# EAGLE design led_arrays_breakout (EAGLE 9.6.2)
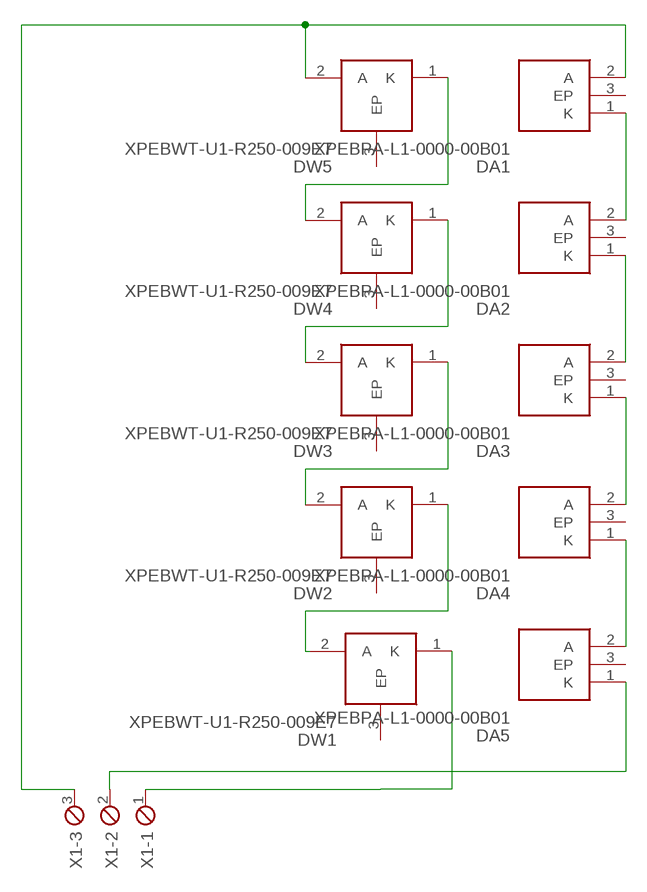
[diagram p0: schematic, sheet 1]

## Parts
DA1  XPEBPA-L1-0000-00B01  [XPEBPAL1000000B01]
DA2  XPEBPA-L1-0000-00B01  [XPEBPAL1000000B01]
DA3  XPEBPA-L1-0000-00B01  [XPEBPAL1000000B01]
DA4  XPEBPA-L1-0000-00B01  [XPEBPAL1000000B01]
DA5  XPEBPA-L1-0000-00B01  [XPEBPAL1000000B01]
DW1  XPEBWT-U1-R250-009E7  [XPEWHTL1000000E01]
DW2  XPEBWT-U1-R250-009E7  [XPEWHTL1000000E01]
DW3  XPEBWT-U1-R250-009E7  [XPEWHTL1000000E01]
DW4  XPEBWT-U1-R250-009E7  [XPEWHTL1000000E01]
DW5  XPEBWT-U1-R250-009E7  [XPEWHTL1000000E01]
X1  MPT3  [3POL254]

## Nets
N$1: DW4.2(A) DW5.1(K)
N$2: DW3.2(A) DW4.1(K)
N$3: DW2.2(A) DW3.1(K)
N$4: DW1.2(A) DW2.1(K)
N$5: DA5.1(K) X1.2
N$6: DW1.1(K) X1.1
N$9: DA1.2(A) DW5.2(A) X1.3
N$24: DA1.1(K) DA2.2(A)
N$25: DA2.1(K) DA3.2(A)
N$26: DA3.1(K) DA4.2(A)
N$27: DA4.1(K) DA5.2(A)
Unconnected: DA1.3(EP) DA2.3(EP) DA3.3(EP) DA4.3(EP) DA5.3(EP) DW1.3(EP) DW2.3(EP) DW3.3(EP) DW4.3(EP) DW5.3(EP)

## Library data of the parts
DA1-DA5 = SamacSys_Parts:XPEBPA-L1-0000-00B01: Cree XPEBPA-L1-0000-00B01, XLamp XP-E2 Series PC Amber LED, 595 nm, Clear, Dome Lens SMD Package Source: Datasheet; DESCRIPTION: Cree XPEBPA-L1-0000-00B01, XLamp XP-E2 Series PC Amber LED, 595 nm, Clear, Dome Lens SMD Package; HEIGHT: 2.53mm; MANUFACTURER_NAME: Wolfspeed; MANUFACTURER_PART_NUMBER: XPEBPA-L1-0000-00B01; MOUSER_PART_NUMBER: 941-XPEBPAL10000B01; MOUSER_PRICE-STOCK: https://www.mouser.co.uk/ProductDetail/Cree-Inc/XPEBPA-L1-0000-00B01?qs=odi%2FggezlBvEJ61b2kTHEA%3D%3D
DW1-DW5 = SamacSys_Parts:XPEBWT-U1-R250-009E7: Cree XPEBWT-U1-R250-009E7, XLamp XP-E2 Series White High-Power LED, 3000K,, Square Lens SMD Package Source: Datasheet; ARROW_PART_NUMBER: XPEBWT-U1-R250-009E7; ARROW_PRICE-STOCK: https://www.arrow.com/en/products/xpebwt-u1-r250-009e7/cree; DESCRIPTION: Cree XPEBWT-U1-R250-009E7, XLamp XP-E2 Series White High-Power LED, 3000K,, Square Lens SMD Package; HEIGHT: mm; MANUFACTURER_NAME: Wolfspeed; MANUFACTURER_PART_NUMBER: XPEBWT-U1-R250-009E7; MOUSER_PART_NUMBER: 941-XPEBWTU1R2509E7; MOUSER_PRICE-STOCK: https://www.mouser.com/Search/Refine.aspx?Keyword=941-XPEBWTU1R2509E7
X1 = con-phoenix-254:MPT3: PHOENIX CONNECTOR; OC_FARNELL: unknown; OC_NEWARK: unknown

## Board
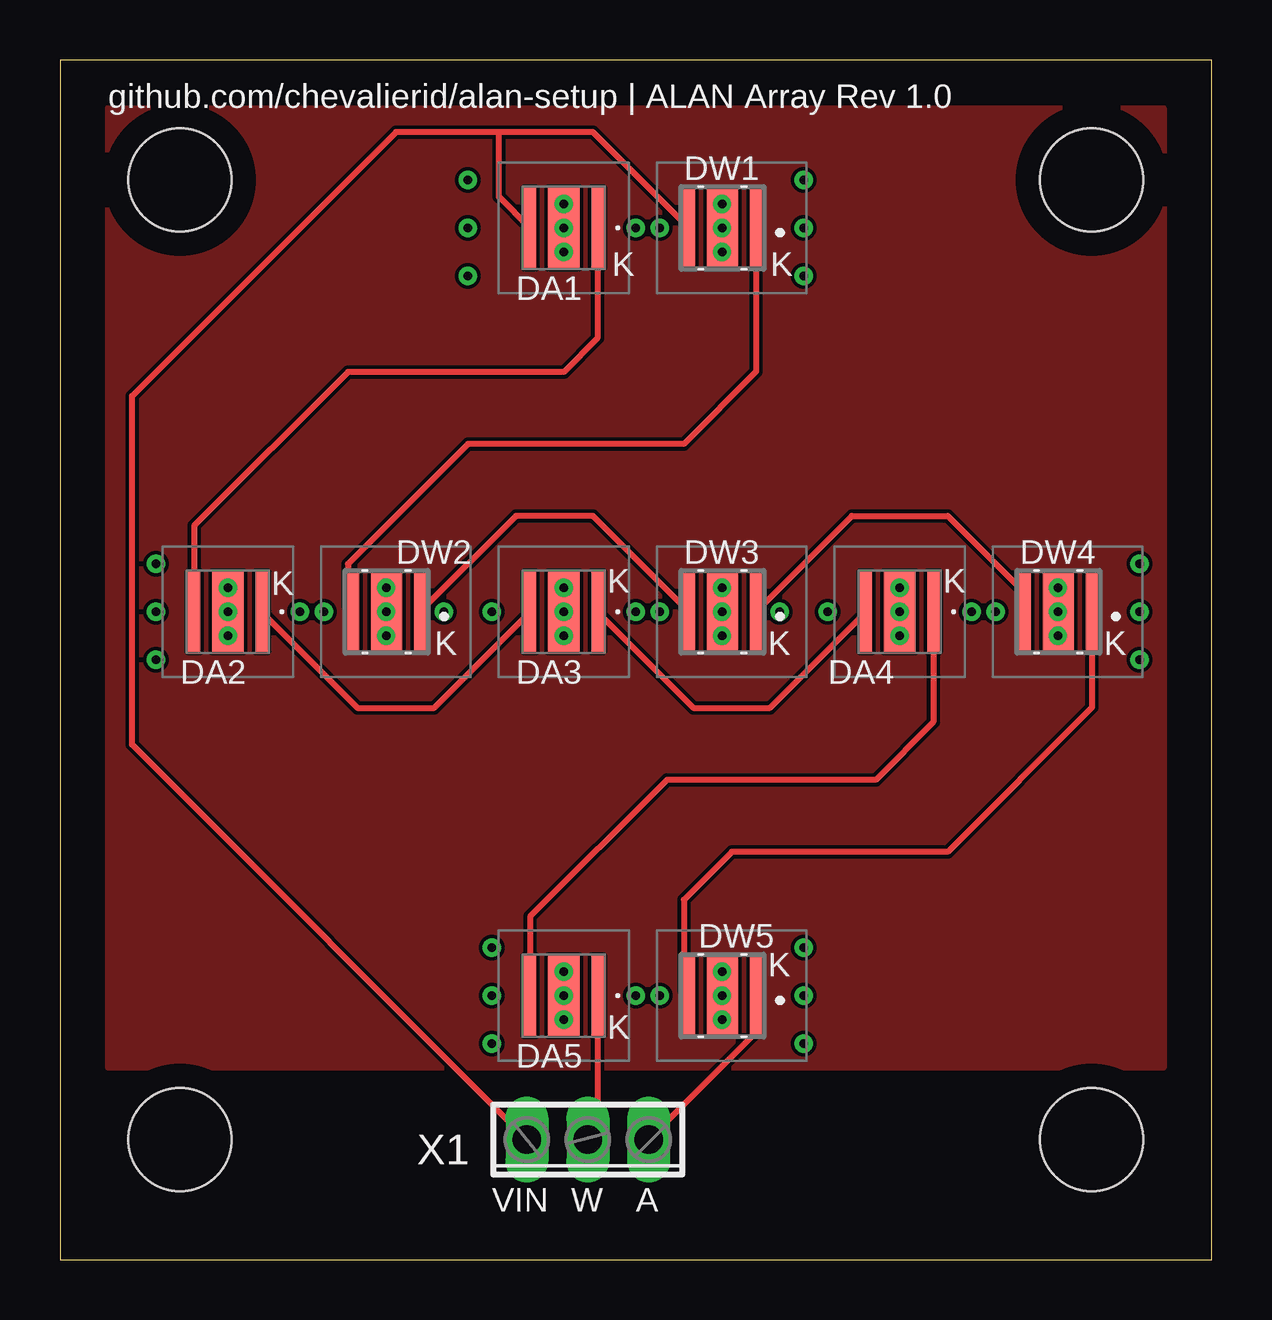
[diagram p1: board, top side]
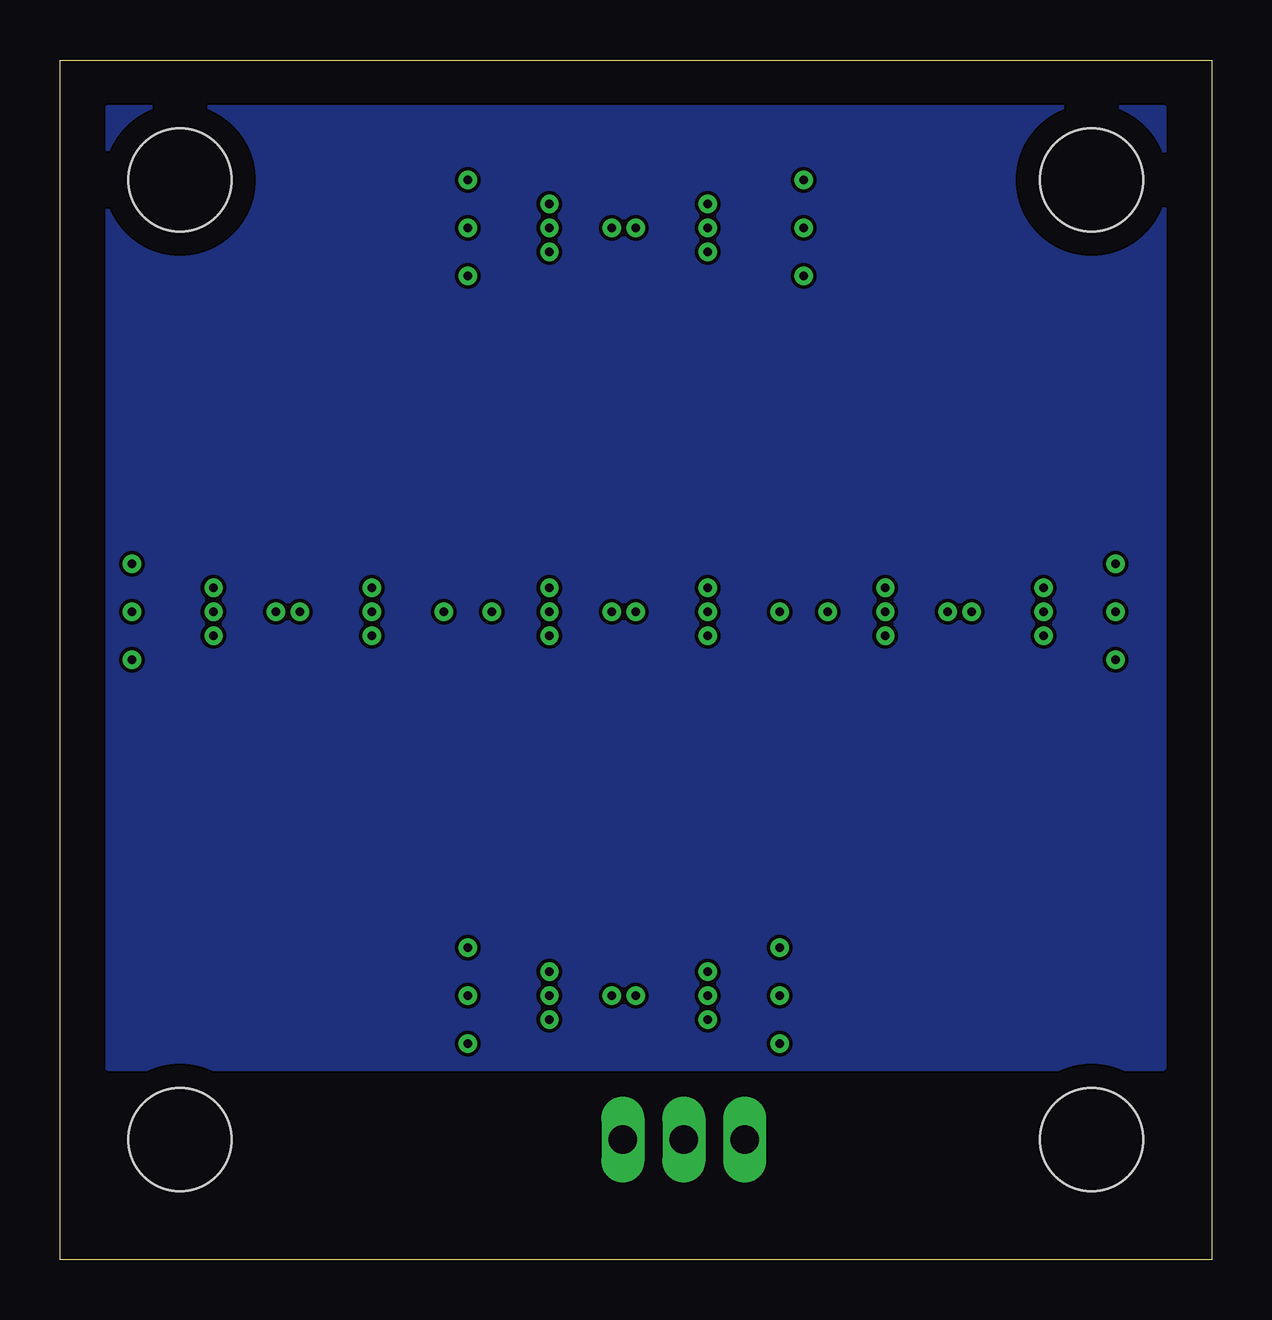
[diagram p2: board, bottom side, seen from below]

Size 48 x 50 mm. Coordinates in mm from the lower left corner, seen from the top.
Outline: 0,0 48,0 48,50 0,50 0,0
Copper layers (1*16): Top 0.035mm / dielectric 1.5mm / Bottom 0.035mm
Design rules "default": minimum track width 6mil, minimum drill 0.35mm, track to track 6mil, track to pad 6mil, pad to pad 6mil, via to via 6mil, smd to smd 6mil, copper to edge 40mil, drill to drill 6mil, minimum pad ring 10mil, minimum via ring 8mil, stop-mask expansion 4mil, vias tented up to drill 0mil, thermal gap 10mil
Holes 4.3 mm at 5,45 43,45 5,5 43,5

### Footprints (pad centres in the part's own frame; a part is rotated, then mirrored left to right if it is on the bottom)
XPEBPAL1000000B01 = smd 0.5 x 3.3: 1 -1.4,0; 2 1.4,0 | smd 1.3 x 3.3: 3 0,0
XPEWHTL1000000E01 = smd 0.5 x 3.3: 1 -1.012,0; 2 1.788,0 | smd 1.3 x 3.3: 3 0.388,0
3POL254 = drill 1.2 long: 1 -2.54,0; 2 0,0; 3 2.54,0

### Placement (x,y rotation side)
DA1  21,43 180 top
DA2  7,27 180 top
DA3  21,27 180 top
DA4  35,27 180 top
DA5  21,11 180 top
DW1  28,11 180 top
DW2  42,27 180 top
DW3  28,27 180 top
DW4  14,27 180 top
DW5  28,43 180 top
X1  22,5 180 top

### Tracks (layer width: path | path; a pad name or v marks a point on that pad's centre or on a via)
HEATSINK_BOTTOM
  pour Bottom: 2,48 46,48 46,8 2,8
HEATSINK_TOP
  pour Top: 2,48 46,48 46,8 2,8
N$1
  Top 0.254: DW4.2 12,27.21 12,29 17,34 26,34 29.01,37.01 DW5.1 29,42.99
N$2
  Top 0.254: DW3.2 22.21,31 19,31 15.01,27.01 DW4.1
N$3
  Top 0.152: 33,30.99 33,31 | 40.21,27.79 DW2.2
  Top 0.254: DW3.1 33,30.99 | 33,31 37,31 40.21,27.79
N$4
  Top 0.254: DW2.1 43.01,23.01 37,17 28,17 26,15 26,11.21 DW1.2
N$5
  Top 0.254: DA5.1 22.4,5.4 X1.2
N$6
  Top 0.254: X1.1 29.01,9.47 DW1.1
N$7  (via drill 0.35)
  other vias: 21,44
N$8  (via drill 0.35)
  other vias: 21,43
N$9
  Top 0.254: X1.3 3,21.46 3,36 14,47 18.3,47 | DW5.2 22.21,47 18.3,47 | DA1.2 18.3,44.3 18.3,47
N$10  (via drill 0.35)
  other vias: 21,42
N$11  (via drill 0.35)
  other vias: 27.6,44
N$12  (via drill 0.35)
  other vias: 27.6,43
N$13  (via drill 0.35)
  other vias: 27.6,42
N$14  (via drill 0.35)
  other vias: 7,28
N$15  (via drill 0.35)
  other vias: 7,27
N$16  (via drill 0.35)
  other vias: 7,26
N$17  (via drill 0.35)
  other vias: 13.6,28
N$18  (via drill 0.35)
  other vias: 13.6,27
N$19  (via drill 0.35)
  other vias: 13.6,26
N$20  (via drill 0.35)
  other vias: 21,28
N$21  (via drill 0.35)
  other vias: 21,27
N$22  (via drill 0.35)
  other vias: 21,26
N$23  (via drill 0.35)
  other vias: 27.6,28
N$24
  Top 0.254: DA1.1 22.4,38.4 21,37 12,37 5.6,30.6 DA2.2
N$25
  Top 0.254: DA2.1 12.4,23 15.6,23 DA3.2
N$26
  Top 0.254: DA3.1 26.4,23 29.6,23 DA4.2
N$27
  Top 0.254: DA4.1 36.4,22.4 34,20 25.3,20 19.6,14.29 DA5.2
N$28  (via drill 0.35)
  other vias: 27.6,27
N$29  (via drill 0.35)
  other vias: 27.6,26
N$30  (via drill 0.35)
  other vias: 35,28
N$31  (via drill 0.35)
  other vias: 35,27
N$32  (via drill 0.35)
  other vias: 35,26
N$33  (via drill 0.35)
  other vias: 41.6,28
N$34  (via drill 0.35)
  other vias: 41.6,27
N$35  (via drill 0.35)
  other vias: 41.6,26
N$36  (via drill 0.35)
  other vias: 21,12
N$37  (via drill 0.35)
  other vias: 21,11
N$38  (via drill 0.35)
  other vias: 21,10
N$39  (via drill 0.35)
  other vias: 27.6,12
N$40  (via drill 0.35)
  other vias: 27.6,11
N$41  (via drill 0.35)
  other vias: 27.6,10
N$42  (via drill 0.35)
  other vias: 17,43
N$43  (via drill 0.35)
  other vias: 17,41
N$44  (via drill 0.35)
  other vias: 24,43
N$45  (via drill 0.35)
  other vias: 25,43
N$46  (via drill 0.35)
  other vias: 31,43
N$47  (via drill 0.35)
  other vias: 31,45
N$48  (via drill 0.35)
  other vias: 4,27
N$49  (via drill 0.35)
  other vias: 10,27
N$50  (via drill 0.35)
  other vias: 11,27
N$51  (via drill 0.35)
  other vias: 4,25
N$52  (via drill 0.35)
  other vias: 18,27
N$53  (via drill 0.35)
  other vias: 16,27
N$54  (via drill 0.35)
  other vias: 24,27
N$55  (via drill 0.35)
  other vias: 25,27
N$56  (via drill 0.35)
  other vias: 30,27
N$57  (via drill 0.35)
  other vias: 4,29
N$58  (via drill 0.35)
  other vias: 32,27
N$59  (via drill 0.35)
  other vias: 38,27
N$60  (via drill 0.35)
  other vias: 39,27
N$61  (via drill 0.35)
  other vias: 45,27
N$62  (via drill 0.35)
  other vias: 45,29
N$63  (via drill 0.35)
  other vias: 45,25
N$64  (via drill 0.35)
  other vias: 18,11
N$65  (via drill 0.35)
  other vias: 18,13
N$66  (via drill 0.35)
  other vias: 18,9
N$67  (via drill 0.35)
  other vias: 31,13
N$68  (via drill 0.35)
  other vias: 31,11
N$69  (via drill 0.35)
  other vias: 31,9
N$70  (via drill 0.35)
  other vias: 24,11
N$71  (via drill 0.35)
  other vias: 25,11
N$72  (via drill 0.35)
  other vias: 31,41
N$73  (via drill 0.35)
  other vias: 17,45

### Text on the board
tPlace: github.com/chevalierid/alan-setup | ALAN Array Rev 1.0 | DW1 | K | K | DA1 | DW2 | DW3 | DW4 | K | K | K | K | K | K | DA2 | DA3 | DA4 | DW5 | K | K | DA5 | VIN | W | A
tStop: K | K | K | K | K | K | K | K | K | K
